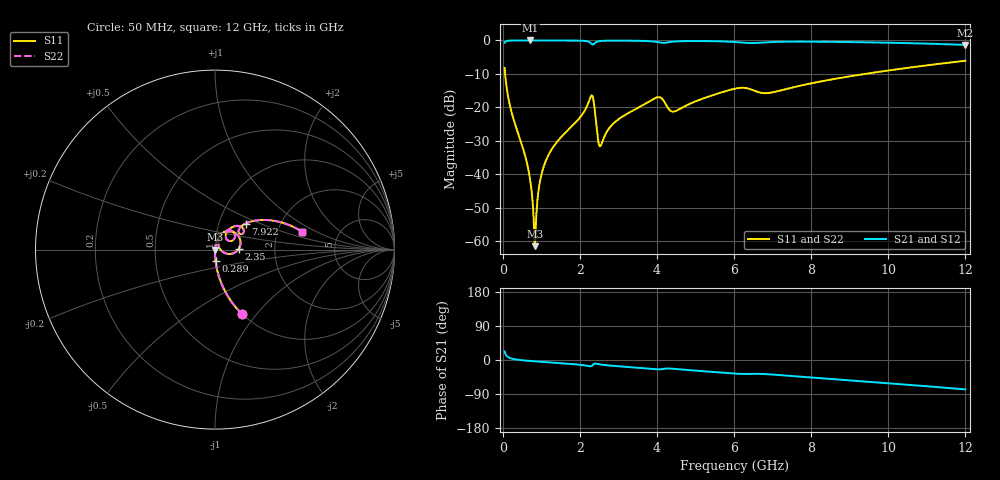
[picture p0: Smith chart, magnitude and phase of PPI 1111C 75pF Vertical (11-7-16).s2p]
# GHz S MA R 50
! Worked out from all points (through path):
!   1601 points, 50 MHz to 12 GHz, reference 50 ohm
!   highest |S21| = -0.01 dB at 714.7 MHz (marker M1); lowest = -1.3 dB at 12 GHz (marker M2)
!   group delay of S21, straight-line fit = 17.9 ps
!   lowest |S11| = -61.5 dB at 834.2 MHz (marker M3), VSWR 1.00, Z = 50.1 - j0.00934 ohm
!   |S11| at or under -10 dB: 63.08 MHz to 9.404 GHz (9.341 GHz wide, 197 % of centre)
!   |S22| runs from -61.5 to -6.1 dB; largest |S21 - S12| = 0
!   S11 on the Smith chart (normalised r, x): 50 MHz: 1.00, -0.84; 289 MHz: 1.00, -0.13; 2.35 GHz: 1.30, +0.01; 7.922 GHz: 1.34, +0.41; 12 GHz: 2.76, +0.72
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0.05  0.388 -67.3  0.9214 22.6  0.9214 22.6  0.388 -67.3
0.289  0.06437 -87.1  0.9974 2.5  0.9974 2.5  0.06437 -87.1
0.5802812  0.01905 -89.3  0.9991 -1.4  0.9991 -1.4  0.01905 -89.3
0.7147187  0.00808 -87.1  0.9991 -2.6  0.9991 -2.6  0.00808 -87.1
0.796875  0.00255 -74.5  0.9991 -3.3  0.9991 -3.3  0.00255 -74.5
0.8342188  0.0008404 -6.4  0.9991 -3.6  0.9991 -3.6  0.0008404 -6.4
0.9835938  0.008702 79.3  0.999 -4.7  0.999 -4.7  0.008702 79.3
1.147906  0.01733 80.8  0.9988 -5.9  0.9988 -5.9  0.01733 80.8
2.044156  0.0753 72.3  0.9909 -13.0  0.9909 -13.0  0.0753 72.3
2.283156  0.1442 40.5  0.9143 -16.7  0.9143 -16.7  0.1442 40.5
2.350375  0.132 1.5  0.8709 -11.7  0.8709 -11.7  0.132 1.5
2.469875  0.03366 -6.7  0.9663 -10.6  0.9663 -10.6  0.03366 -6.7
2.537094  0.02652 32.8  0.9808 -11.9  0.9808 -11.9  0.02652 32.8
2.955344  0.06311 69.1  0.9926 -16.1  0.9926 -16.1  0.06311 69.1
4.038312  0.142 43.8  0.9387 -24.6  0.9387 -24.6  0.142 43.8
4.441625  0.08647 43.2  0.9621 -23.3  0.9621 -23.3  0.08647 43.2
6.025  0.1901 43.4  0.9468 -35.9  0.9468 -35.9  0.1901 43.4
6.8615  0.1632 35.6  0.9398 -37.5  0.9398 -37.5  0.1632 35.6
7.922063  0.2235 40.5  0.9589 -45.5  0.9589 -45.5  0.2235 40.5
8.019156  0.2296 40.1  0.9582 -46.3  0.9582 -46.3  0.2296 40.1
10.01331  0.3562 27.1  0.9246 -61.4  0.9246 -61.4  0.3562 27.1
12  0.4966 11.5  0.8584 -77.5  0.8584 -77.5  0.4966 11.5
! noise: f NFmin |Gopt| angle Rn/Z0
0.05  0.0003628  0.8629  0.4765  0.0005677
1.372  0.003969  0.6887  5.736  0.002473
2.701  0.01465  0.8219  11.43  0.01709
4.031  0.04448  0.9091  16.98  0.1053
5.36  0.02527  0.8018  22.26  0.02547
6.682  0.06305  0.8973  27.71  0.1265
8.012  0.03303  0.7833  32.56  0.02887
9.341  0.02947  0.7313  37.09  0.0197
10.67  0.03019  0.7113  41.46  0.01809
12  0.03243  0.7071  45.68  0.01858
